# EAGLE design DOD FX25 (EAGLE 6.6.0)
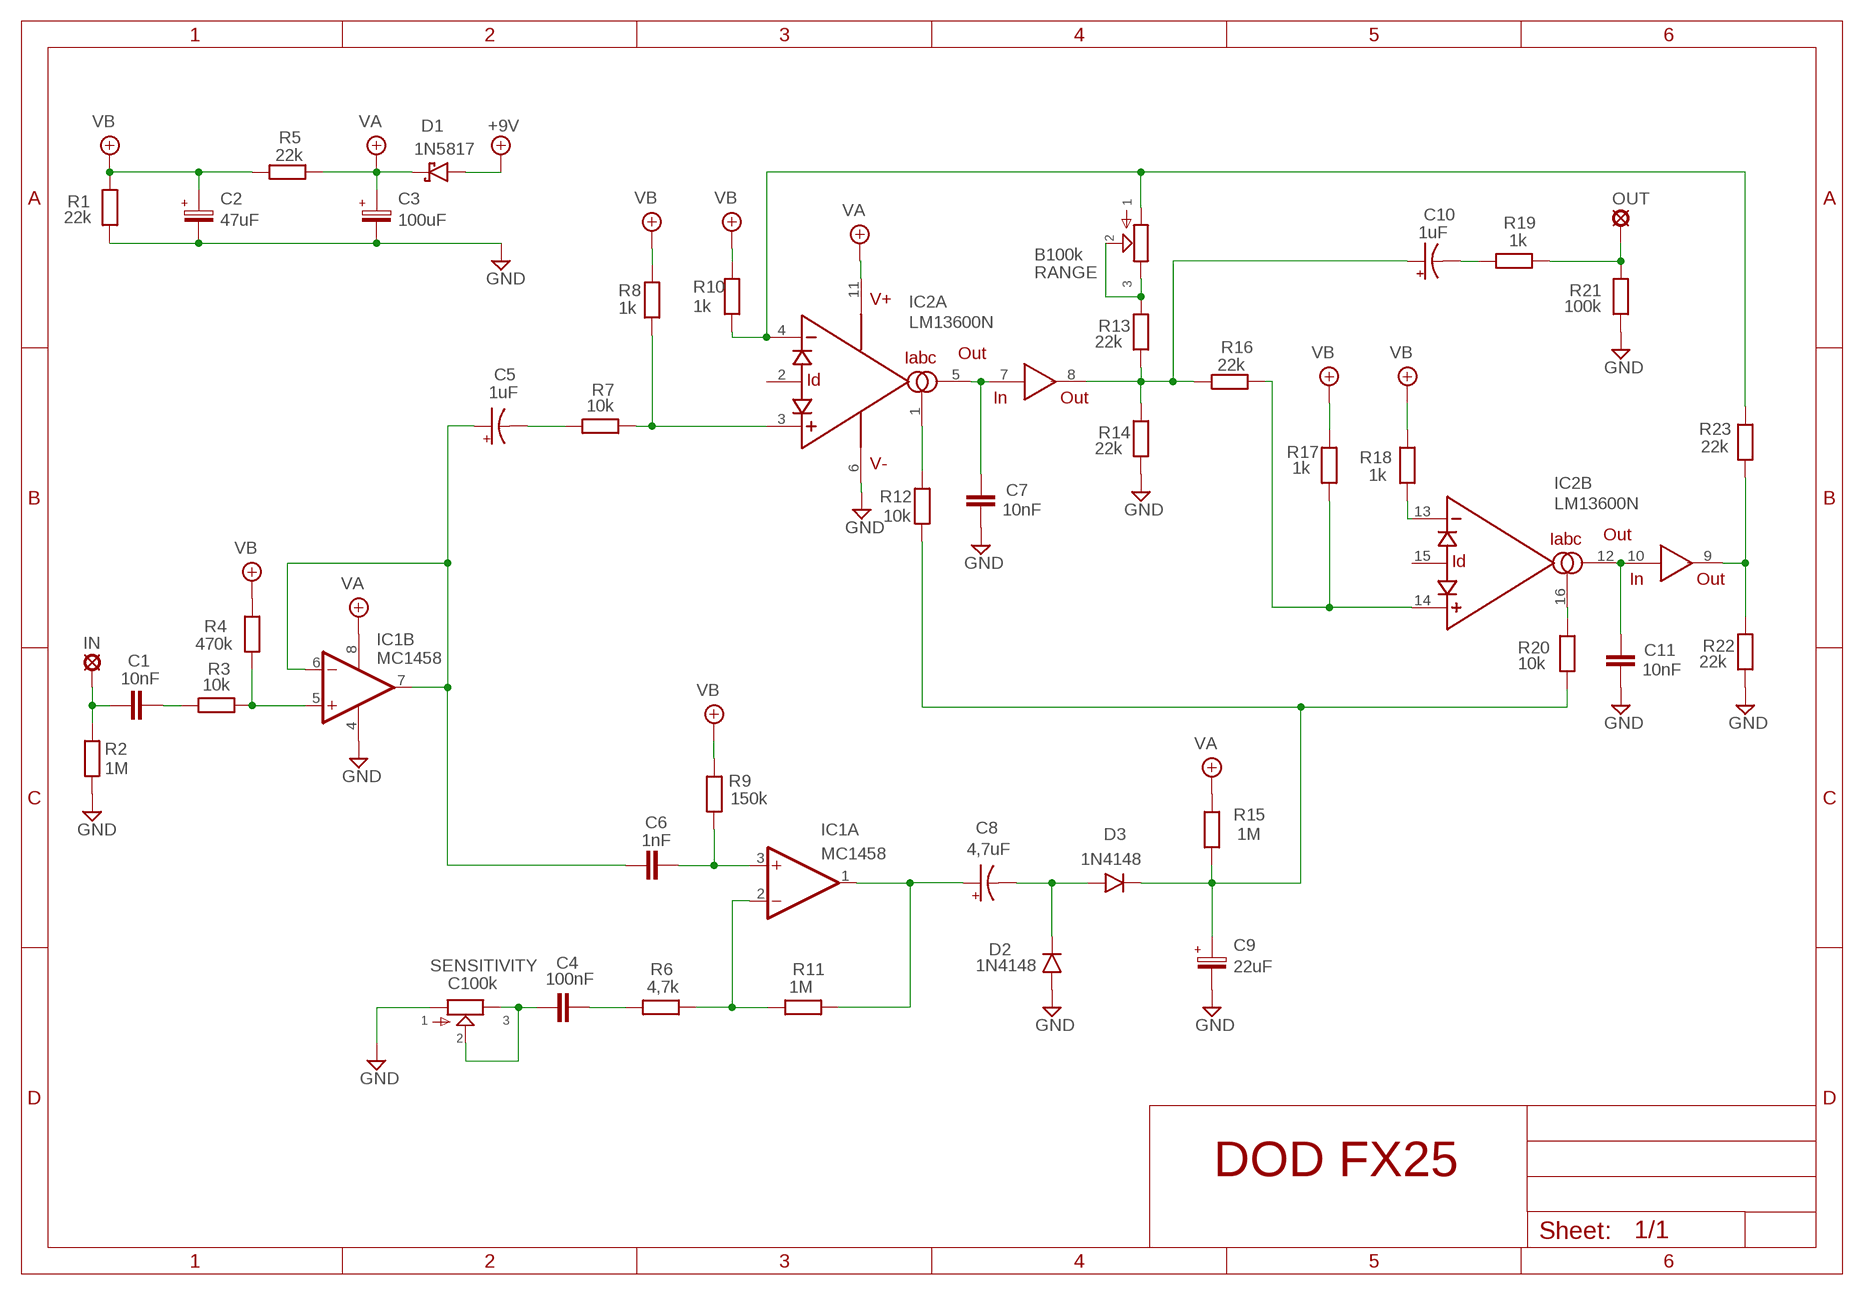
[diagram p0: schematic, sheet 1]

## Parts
+9V  +9V  +9V(T)1  [ROUND]
C1  10nF  1NF-15NF  [3,5MM]
C2  47uF  063-EU  [063_025]
C3  100uF  063-EU  [063_025]
C4  100nF  100NF-220NF  [7,5MM]
C5  1uF  044A1  [044A]
C6  1nF  1NF-15NF  [3,5MM]
C7  10nF  1NF-15NF  [3,5MM]
C8  4,7uF  044A1  [044A]
C9  22uF  063-EU  [063_025]
C10  1uF  044A1  [044A]
C11  10nF  1NF-15NF  [3,5MM]
D1  1N5817  [DO41-3]
D2  1N4148  1N4148-3  [DO35-3]
D3  1N4148  1N4148-3  [DO35-3]
GND  GND  GND(T)1  [ROUND]
GND1  GND  GND(T)1  [ROUND]
IC1  MC1458  TL072P  [DIL08]
IC2  LM13600N  [DIL16]
IN  MCS10B  [MCS10B]
OUT  MCS10B  [MCS10B]
R1  22k  6MM-EU3  [R0207/3]
R2  1M  6MM-EU3  [R0207/3]
R3  10k  6MM-EU3  [R0207/3]
R4  470k  6MM-EU3  [R0207/3]
R5  22k  6MM-EU3  [R0207/3]
R6  4,7k  6MM-EU3  [R0207/3]
R7  10k  6MM-EU3  [R0207/3]
R8  1k  6MM-EU3  [R0207/3]
R9  150k  6MM-EU3  [R0207/3]
R10  1k  6MM-EU3  [R0207/3]
R11  1M  6MM-EU3  [R0207/3]
R12  10k  6MM-EU3  [R0207/3]
R13  22k  6MM-EU3  [R0207/3]
R14  22k  6MM-EU3  [R0207/3]
R15  1M  6MM-EU3  [R0207/3]
R16  22k  6MM-EU3  [R0207/3]
R17  1k  6MM-EU3  [R0207/3]
R18  1k  6MM-EU3  [R0207/3]
R19  1k  6MM-EU3  [R0207/3]
R20  10k  6MM-EU3  [R0207/3]
R21  100k  6MM-EU3  [R0207/3]
R22  22k  6MM-EU3  [R0207/3]
R23  22k  6MM-EU3  [R0207/3]
RANGE  B100k  POT-EU16MM  [16MM]
SENSITIVITY  C100k  POT-EU16MM  [16MM]

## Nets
+9V: +9V.1(+9V) D1.A
GND: C2.- C3.- C7.2 C9.- C11.2 D2.A GND1.1(GND) GND.1(GND) IC1.4(P:V-) IC2.6(V-) R1.1 R2.1 R14.1 R21.1 R22.1 SENSITIVITY.1
N$1: C5.1(+) C6.1 IC1.6(B:-IN) IC1.7(B:OUT)
N$2: IC2.3(A:+IN) R7.2 R8.2
N$3: C5.2(-) R7.1
N$4: IC2.4(A:-IN) R10.2 R23.2 RANGE.1
N$5: IC1.5(B:+IN) R3.2 R4.2
N$6: IC2.1(A:IABC) R12.1
N$7: C1.2 R3.1
N$8: C1.1 IN.MP R2.2
N$9: C7.1 IC2.5(A:OUT) IC2.7(IN)
N$10: IC2.16(B:IABC) R20.1
N$11: R13.2 RANGE.2 RANGE.3
N$12: C4.P$1 SENSITIVITY.2 SENSITIVITY.3
N$13: C10.1(+) IC2.8(OUT) R13.1 R14.2 R16.1
N$14: C10.2(-) R19.1
N$15: OUT.MP R19.2 R21.2
N$16: IC2.14(B:+IN) R16.2 R17.2
N$17: IC2.13(B:-IN) R18.2
N$18: C11.1 IC2.10(IN) IC2.12(B:OUT)
N$19: IC2.9(OUT) R22.2 R23.1
N$20: C8.1(+) IC1.1(A:OUT) R11.2
N$21: IC1.2(A:-IN) R6.2 R11.1
N$22: C6.2 IC1.3(A:+IN) R9.1
N$23: C4.P$2 R6.1
N$25: C8.2(-) D2.C D3.A
N$26: C9.+ D3.C R12.2 R15.1 R20.2
VA: C3.+ D1.C IC1.8(P:V+) IC2.11(V+) R5.2 R15.2
VB: C2.+ R1.2 R4.1 R5.1 R8.1 R9.2 R10.1 R17.1 R18.1
Unconnected: IC2.2(A:ID) IC2.15(B:ID)

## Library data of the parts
+9V = gm-supply:+9V(T): +9V Voltage Supply
C1 C6 C7 C11 = Mylar Kondensaattorit:1NF-15NF: 1nF-15nF
C2 C3 C9 = Elektrolyytit:063-EU
C4 = Mylar Kondensaattorit:100NF-220NF: 100nF-220nF
C5 C8 C10 = gm-caps-tant:044A: .1 - 1.5µF
D1 = Diodit:1N5817
D2 D3 = Diodit:1N4148: Fast Switching Diode
GND GND1 = gm-supply:GND(T): Ground
IC1 = Operaatiovahvistimet:TL072: OP AMP
IC2 = synthdiy:LM13600: National Dual OTA with buffers.
IN OUT = Padit:MCS10B: SOLDER PAD
R1-R23 = Vastukset:6MM-EU: 6mm Resistors (European schematic symbol)
RANGE SENSITIVITY = gm-pots:POT-EU

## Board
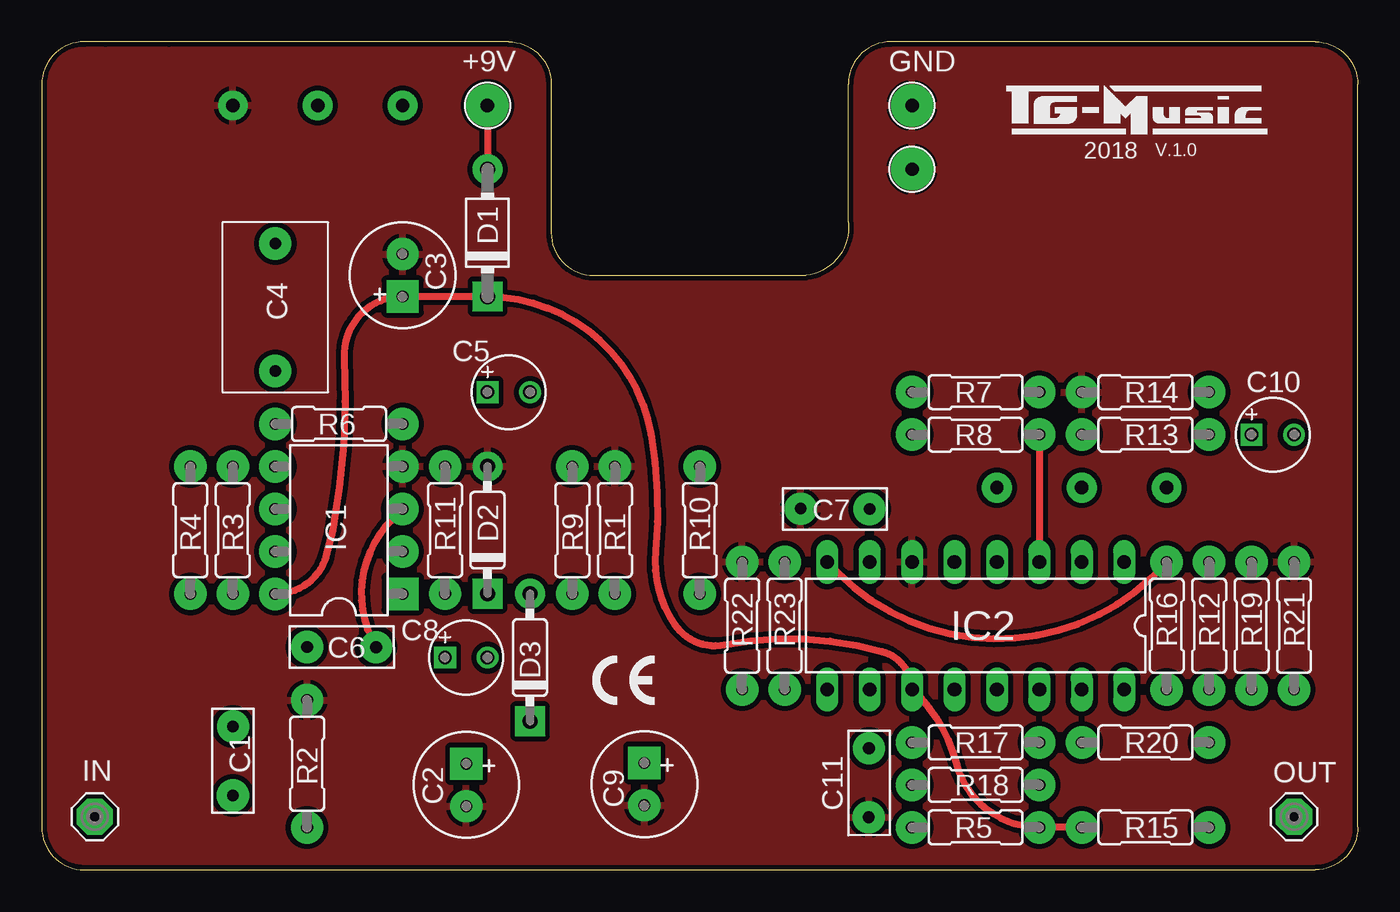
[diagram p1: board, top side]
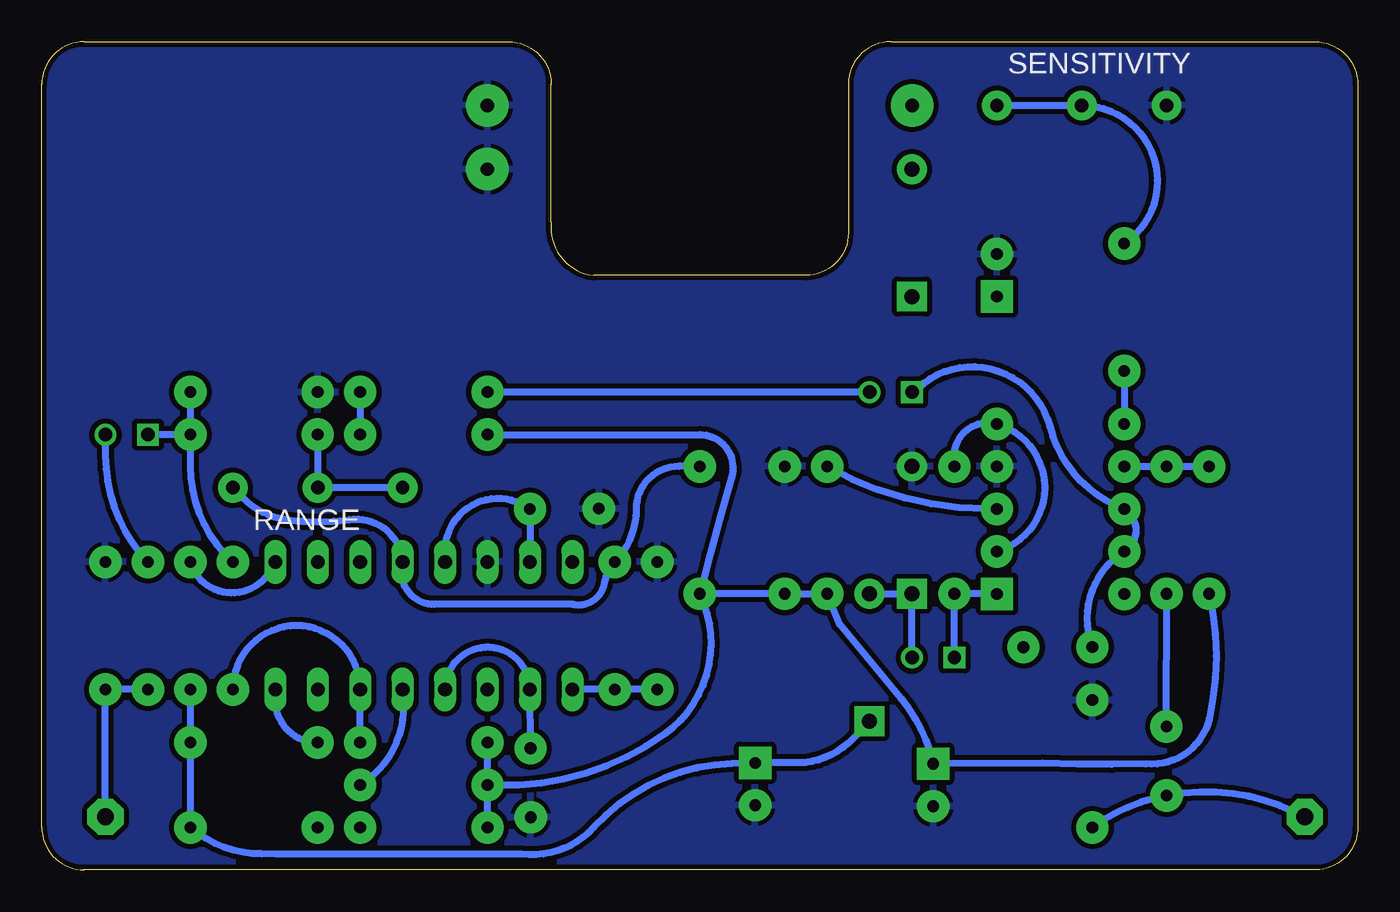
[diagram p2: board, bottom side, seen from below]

Size 78.74 x 49.53 mm. Coordinates in mm from the lower left corner, seen from the top.
Outline: 7.62,49.53 3.81,49.53
Outline: 78.74,2.54 78.74,46.99 arc90 76.2,49.53 50.8,49.53 arc90 48.26,46.99 48.26,38.73 arc-90 45.72,35.56 33.02,35.56 arc-90 30.48,38.1 30.48,46.99 arc90 27.94,49.53 2.54,49.53 arc90 0,46.99 0,2.54 arc90 2.54,0 76.2,0 arc90 78.74,2.54
Copper layers (1*16): Top 0.035mm / dielectric 1.5mm / Bottom 0.035mm
Design rules "ITEADstudio": minimum track width 10mil, minimum drill 12mil, track to track 12mil, track to pad 12mil, pad to pad 12mil, via to via 12mil, smd to smd 0mil, copper to edge 12mil, drill to drill 12mil, minimum pad ring 10mil, minimum via ring 6mil, stop-mask expansion 4mil, vias tented up to drill 100mil, thermal gap 10mil

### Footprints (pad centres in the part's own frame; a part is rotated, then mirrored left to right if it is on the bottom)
ROUND = drill 0.8 pad 2.54: 1 0,0
3,5MM = drill 0.7 pad 1.93: 1 -1.905,0; 2 2.221,-0.016
063_025 = drill 0.7 pad 1.93 square: + -1.27,0 | drill 0.7 pad 1.93: - 1.27,0
7,5MM = drill 0.7 pad 1.93: P$1 -3.81,0; P$2 3.81,0
044A = drill 0.8 square: 1 -1.27,0 | drill 0.8: 2 1.27,0
DO41-3 = drill 0.9 pad 1.778: A 3.81,0 | drill 0.9 pad 1.778 square: C -3.81,0
DO35-3 = drill 0.9 pad 1.778: A 3.81,0 | drill 0.9 pad 1.778 square: C -3.81,0
DIL08 = drill 0.7 pad 1.93 square: 1 -3.81,-3.81 | drill 0.7 pad 1.93: 2 -1.27,-3.81; 3 1.27,-3.81; 4 3.81,-3.81; 5 3.81,3.81; 6 1.27,3.81; 7 -1.27,3.81; 8 -3.81,3.81
DIL16 = drill 0.813 long: 1 -8.89,-3.81; 2 -6.35,-3.81; 3 -3.81,-3.81; 4 -1.27,-3.81; 5 1.27,-3.81; 6 3.81,-3.81; 7 6.35,-3.81; 8 8.89,-3.81; 9 8.89,3.81; 10 6.35,3.81; 11 3.81,3.81; 12 1.27,3.81; 13 -1.27,3.81; 14 -3.81,3.81; 15 -6.35,3.81; 16 -8.89,3.81
MCS10B = drill 1.016 pad 2.159 octagon: MP 0,0
R0207/3 = drill 0.7 pad 1.93: 1 -3.81,0; 2 3.81,0
16MM = drill 0.8 pad 1.778: 1 5.08,0; 2 0,0; 3 -5.08,0

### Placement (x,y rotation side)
+9V  26.67,45.72 0 top
C1  11.43,6.35 90 top
C2  25.4,5.08 270 top
C3  21.59,35.56 90 top
C4  13.97,33.66 270 top
C5  27.94,28.57 0 top
C6  17.78,13.34 0 top
C7  47.62,21.59 180 top
C8  25.4,12.7 0 top
C9  36.05,5.13 270 top
C10  73.66,26.04 0 top
C11  49.5,5.37 270 top
D1  26.67,38.1 90 top
D2  26.67,20.32 90 top
D3  29.21,12.7 90 top
GND  52.07,45.72 0 top
GND1  52.07,41.91 0 top
IC1  17.78,20.32 90 top
IC2  55.88,14.61 180 top
IN  3.17,3.17 0 top
OUT  74.93,3.17 0 top
R1  34.29,20.32 270 top
R2  15.88,6.35 270 top
R3  11.43,20.32 90 top
R4  8.89,20.32 90 top
R5  55.88,2.54 0 top
R6  17.78,26.67 0 top
R7  55.88,28.57 0 top
R8  55.88,26.04 0 top
R9  31.75,20.32 270 top
R10  39.37,20.32 90 top
R11  24.13,20.32 270 top
R12  69.85,14.61 270 top
R13  66.04,26.04 180 top
R14  66.04,28.57 0 top
R15  66.04,2.54 180 top
R16  67.31,14.61 270 top
R17  55.88,7.62 0 top
R18  55.88,5.08 0 top
R19  72.39,14.61 270 top
R20  66.04,7.62 0 top
R21  74.93,14.61 270 top
R22  41.91,14.61 270 top
R23  44.45,14.61 90 top
RANGE  62.23,22.86 180 bottom
SENSITIVITY  16.51,45.72 0 bottom

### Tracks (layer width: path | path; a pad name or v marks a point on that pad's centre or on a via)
+9V
  Top 0.406: +9V.1 D1.A
GND
  pour Bottom: 0,2.54 0,46.99 arc-90 2.54,49.53 27.94,49.53 arc-90 30.48,46.99 30.48,38.1 arc90 33.02,35.56 45.72,35.56 arc90 48.26,38.1 48.26,46.99 arc-90 50.8,49.53 76.2,49.53 arc-90 78.74,46.99 78.74,2.54 arc-90 76.2,0 2.54,0 arc-90
  pour Top: 0,2.54 0,46.99 arc-90 2.54,49.53 27.94,49.53 arc-90 30.48,46.99 30.48,38.1 arc90 33.02,35.56 45.72,35.56 arc90 48.26,38.1 48.26,46.99 arc-90 50.8,49.53 76.2,49.53 arc-90 78.74,46.99 78.74,2.54 arc-90 76.2,0 2.54,0 arc-90
N$1
  Bottom 0.406: C5.1 25.97,29.11 arc113 18.43,26.53 arc-55 IC1.6 arc117 IC1.7 arc-80 C6.1
N$2
  Top 0.406: R8.2 IC2.3
  Bottom 0.406: R7.2 R8.2
N$3
  Bottom 0.406: C5.2 R7.1
N$4
  Bottom 0.406: R10.2 40.64,24.13 arc-90 43.18,21.59 arc44 R23.2 arc-34 45.09,17.14 arc94 46.99,15.88 55.24,15.88 arc106 IC2.4 arc-94 60.33,20.95 arc16 64.14,20.95 arc37 66.67,22.23 RANGE.1
N$5
  Bottom 0.406: IC1.5 R3.2 arc0 R4.2
N$6
  Bottom 0.406: IC2.1 65.12,17.83 arc132 R12.1
N$7
  Bottom 0.406: C1.2 R3.1
N$8
  Bottom 0.406: IN.MP 3.73,3.44 arc-36 C1.1 arc-25 R2.2
N$9
  Bottom 0.406: IC2.7 C7.1 arc-127 54.61,19.05 IC2.5
N$10
  Bottom 0.406: IC2.16 64.77,10.16 arc-90 R20.1
N$11
  Bottom 0.406: RANGE.3 RANGE.2 R13.2
N$12
  Bottom 0.406: SENSITIVITY.3 SENSITIVITY.2 arc146 C4.P$1
N$13
  Top 0.406: IC2.8 47.62,17.78 arc94 R16.1
  Bottom 0.406: R14.2 R13.1 | R13.1 C10.1 | R13.1 69.85,24.13 arc-48 R16.1
N$14
  Bottom 0.406: C10.2 74.93,24.77 arc-44 R19.1
N$15
  Bottom 0.406: R19.2 R21.2 OUT.MP
N$16
  Bottom 0.406: R17.2 IC2.14 arc-180 R16.2
N$17
  Bottom 0.406: IC2.13 57.11,9.95 arc61 R18.2
N$18
  Bottom 0.406: C11.1 IC2.10 arc-179 IC2.12
N$19
  Bottom 0.406: R22.2 R23.1 IC2.9
N$20
  Bottom 0.406: IC1.1 R11.2 C8.1
N$21
  Bottom 0.406: R11.1 24.13,24.77 arc106 R6.2 arc147 IC1.2
N$22
  Top 0.406: IC1.3 20.95,20.95 arc76 C6.2
  Bottom 0.406: IC1.3 22.23,21.59 arc29 R9.1
N$23
  Bottom 0.406: C4.P$2 R6.1
N$25
  Bottom 0.406: C8.2 D2.C D3.A
N$26
  Bottom 0.406: D3.C 30.18,7.86 arc39 33.05,6.41 36.05,6.41 C9.+ 37.47,6.35 arc-46 45.72,2.54 arc55 50.02,0.95 64.74,0.95 65.55,0.95 arc40 R15.1 R20.2 R12.2
VA
  Top 0.406: IC1.8 arc77 17.03,18.85 17.39,20.3 arc14 18.09,30.61 arc-93 C3.+ D1.C arc-80 36.45,26.05 arc-15 36.72,19.08 arc40 37.87,14.68 arc66 40.84,13.46 arc-27 50.29,13.06 arc-72 IC2.11 arc-33 54.75,6.36 arc75 R5.2 R15.2
VB
  Bottom 0.406: R4.1 arc25 8.89,9.05 arc83 12.68,6.35 arc4 18.85,6.38 C2.+ arc-26 27.34,10.26 31.01,14.72 R9.2 | R9.2 | R9.2 R1.2 R10.1 | R8.1 39.37,26.04 arc106 37.47,23.5 arc-2 R10.1 | R5.1 R18.1 | R18.1 R17.1 | R18.1 50.16,5.08 arc-33 41.47,8.13 arc-81 R10.1

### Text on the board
tNames: 2018 | V.1.0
